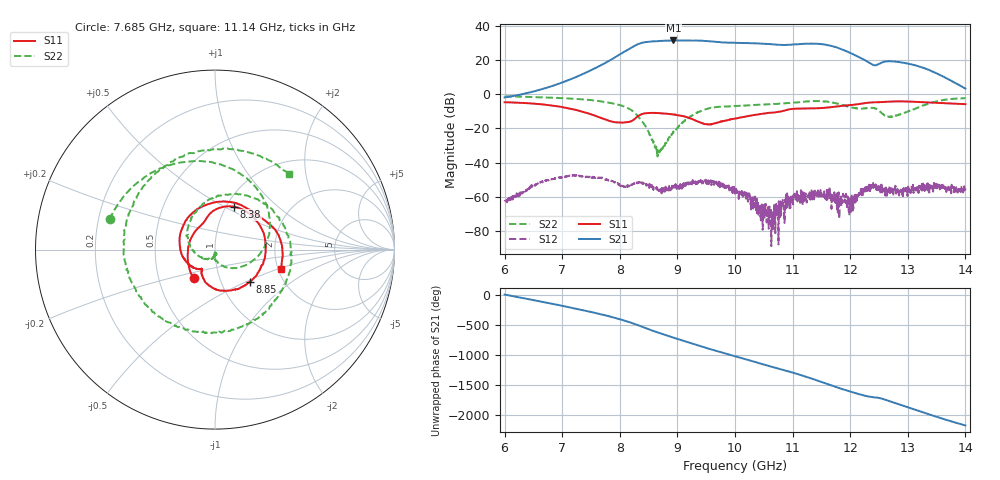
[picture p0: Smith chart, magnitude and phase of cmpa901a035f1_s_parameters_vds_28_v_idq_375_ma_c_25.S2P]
!Keysight Technologies,E5071C,MY46110325,B.14.03
!Date: Wed Mar 10 11:02:29 2021
!Data & Calibration Information:
!Freq	S11:SOLT2(ON)	S21:SOLT2(ON)	S12:SOLT2(ON)	S22:SOLT2(ON)
!PortZ  Port1:50+j0  Port2:50+j0
!Above PortZ is port z conversion or system Z0 setting when saving the data.
!When reading, reference impedance value at option line is always used.
# Hz S dB R 50
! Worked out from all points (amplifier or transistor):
!   1601 points, 6 GHz to 14 GHz, reference 50 ohm
!   highest |S21| = 31.5 dB at 8.93 GHz (marker M1)
!   |S21| within 3 dB of that: 8.265 GHz to 11.64 GHz (3.374 GHz wide, 33.9 % of centre)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
!   unconditionally stable (mu >= 1): start of sweep to end of sweep
!   at 7.33 GHz: K = 15.08, MAG = 14.9 dB, |S12| = -47.9 dB
!   at 10 GHz: K = 9.93, MAG = 31.2 dB, |S12| = -58.3 dB
!   at 14 GHz: K = 59.62, MAG = 8.6 dB, |S12| = -55.3 dB
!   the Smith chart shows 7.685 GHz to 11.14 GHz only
!   S11 on the Smith chart (normalised r, x): 7.685 GHz: 0.75, -0.25; 8.38 GHz: 1.09, +0.56; 8.85 GHz: 1.37, -0.53; 11.14 GHz: 2.08, -0.52
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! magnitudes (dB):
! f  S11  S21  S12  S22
! 6 GHz  -4.7  -1.9  -62.0  -1.2
! 6.705 GHz  -6.1  3.5  -50.6  -1.9
! 7.335 GHz  -10.0  11.5  -48.2  -3.0
! 7.685 GHz  -14.0  17.2  -49.0  -4.3
! 8.095 GHz  -16.5  25.2  -54.2  -7.4
! 8.38 GHz  -11.7  30.1  -51.8  -15.5
! 8.67 GHz  -11.0  31.2  -56.5  -34.6
! 8.85 GHz  -11.5  31.4  -56.4  -25.6
! 8.93 GHz  -11.8  31.5  -54.2  -22.4
! 9.395 GHz  -16.5  31.3  -51.5  -10.1
! 10 GHz  -14.3  30.1  -58.3  -6.9
! 10.22 GHz  -12.8  30.0  -60.5  -6.5
! 10.45 GHz  -11.6  29.7  -71.4  -6.1
! 10.62 GHz  -10.8  29.3  -66.8  -5.9
! 10.9 GHz  -9.1  28.9  -58.1  -5.2
! 11.14 GHz  -8.3  29.4  -56.2  -4.6
! 11.34 GHz  -8.3  29.6  -59.5  -4.0
! 12.02 GHz  -6.3  24.0  -68.9  -7.6
! 12.37 GHz  -4.8  17.7  -54.1  -8.0
! 12.67 GHz  -4.4  19.3  -56.7  -13.2
! 13.27 GHz  -4.7  15.5  -52.4  -6.6
! 14 GHz  -5.8  3.3  -55.3  -2.3
